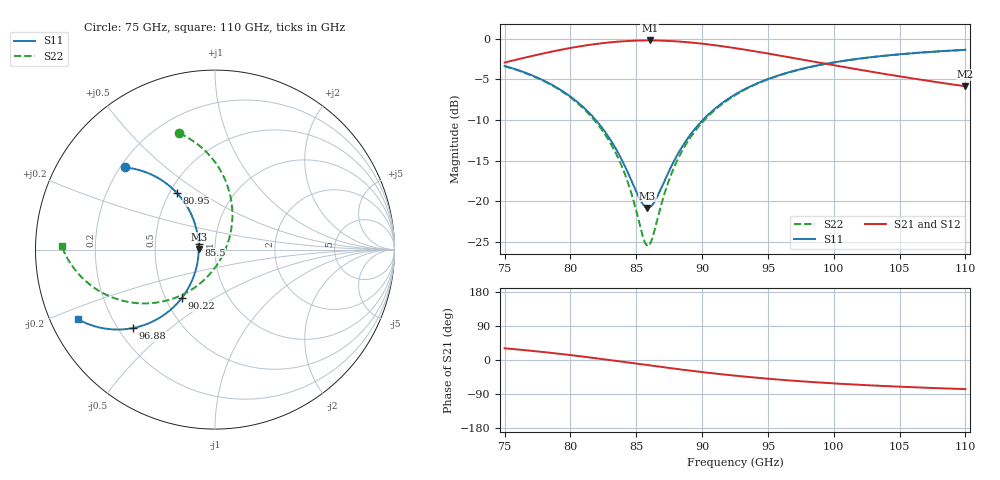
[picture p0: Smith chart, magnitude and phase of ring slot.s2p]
!Created with skrf (http://scikit-rf.org).
# GHz S RI R 50.0
!freq ReS11 ImS11 ReS21 ImS21 ReS12 ImS12 ReS22 ImS22
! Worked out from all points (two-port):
!   201 points, 75 GHz to 110 GHz, reference 50 ohm
!   highest |S21| = -0.20 dB at 86.03 GHz (marker M1); lowest = -5.8 dB at 110 GHz (marker M2)
!   |S21| within 3 dB of the highest: start of sweep to 99.82 GHz
!   lowest |S11| = -20.8 dB at 85.85 GHz (marker M3), VSWR 1.20, Z = 41.7 + j0.293 ohm
!   |S11| at or under -10 dB: 81.92 GHz to 90.06 GHz (8.137 GHz wide, 9.46 % of centre)
!   |S22| runs from -25.6 to -1.4 dB; largest |S21 - S12| = 0
!   S11 on the Smith chart (normalised r, x): 75 GHz: 0.22, +0.37; 80.95 GHz: 0.54, +0.40; 85.5 GHz: 0.83, +0.05; 90.22 GHz: 0.61, -0.36; 96.88 GHz: 0.26, -0.38; 110 GHz: 0.08, -0.24
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75  -0.5037 0.4578  0.6135 0.3668  0.6135 0.3668  -0.1996 0.6483
77.975  -0.3594 0.4205  0.7606 0.2912  0.7606 0.2912  -0.0515 0.5471
80.95  -0.2128 0.316  0.8943 0.142  0.8943 0.142  0.0646 0.3689
82.35  -0.1558 0.2407  0.9378 0.0461  0.9378 0.0461  0.0921 0.2618
83.575  -0.1186 0.1632  0.9594 -0.0473  0.9594 -0.0473  0.096 0.1616
84.45  -0.1011 0.1032  0.9637 -0.117  0.9637 -0.117  0.0861 0.0895
85.5  -0.0913 0.0285  0.9562 -0.2008  0.9562 -0.2008  0.0603 0.00578
85.85  -0.0908 0.00348  0.9506 -0.2282  0.9506 -0.2282  0.0485 -0.0208
86.025  -0.0911 -0.00899  0.9473 -0.2418  0.9473 -0.2418  0.042 -0.0338
86.2  -0.0917 -0.0214  0.9436 -0.2552  0.9436 -0.2552  0.0352 -0.0466
86.725  -0.0955 -0.0583  0.9304 -0.2945  0.9304 -0.2945  0.0126 -0.0834
87.425  -0.1052 -0.1061  0.9083 -0.3444  0.9083 -0.3444  -0.0217 -0.1285
88.125  -0.1195 -0.1516  0.8815 -0.3906  0.8815 -0.3906  -0.0602 -0.1685
89  -0.1432 -0.2044  0.8428 -0.4425  0.8428 -0.4425  -0.1127 -0.211
90.225  -0.1848 -0.2692  0.7815 -0.5032  0.7815 -0.5032  -0.1909 -0.2557
92.5  -0.2772 -0.359  0.6586 -0.5793  0.6586 -0.5793  -0.3371 -0.2965
94.425  -0.3591 -0.4063  0.5573 -0.6114  0.5573 -0.6114  -0.4499 -0.2966
96.875  -0.4565 -0.4371  0.443 -0.6219  0.443 -0.6219  -0.5702 -0.267
98.45  -0.5123 -0.4444  0.38 -0.6167  0.38 -0.6167  -0.6331 -0.2375
101.25  -0.5966 -0.4423  0.2877 -0.5945  0.2877 -0.5945  -0.72 -0.1756
104.225  -0.6674 -0.428  0.2129 -0.5624  0.2129 -0.5624  -0.7845 -0.1061
110  -0.7631 -0.3882  0.1161 -0.4967  0.1161 -0.4967  -0.8552 0.021
